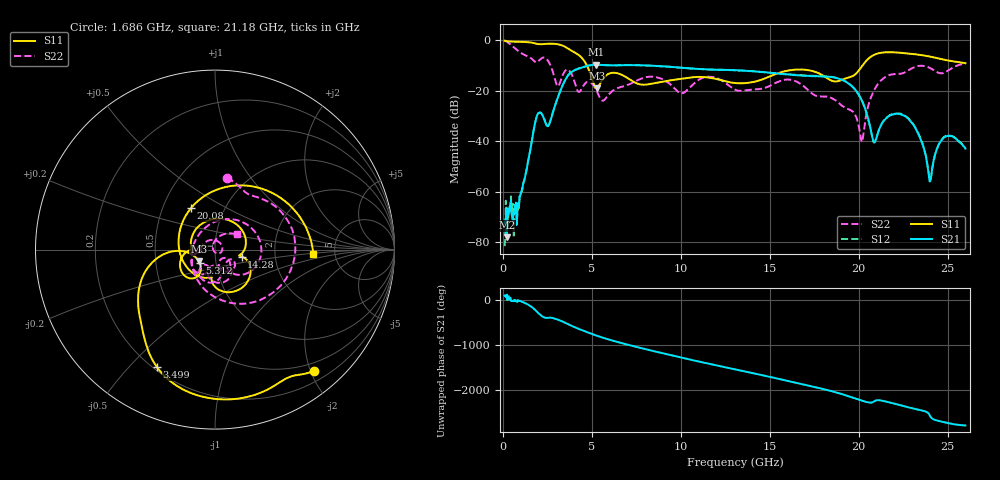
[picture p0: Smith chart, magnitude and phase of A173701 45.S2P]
!  2-Port S-parameters saved by WinCal
! VAR MeasName=S-Parameters (CALIBRATED_DATA) read from VNA (N5245A)
! VAR MeasDate=2017-6-7 10:31:25
! VAR NAME=A173701 45
! VAR FILENAME=A173701 45.S2P
! VAR DATE=2017-6-7 10:31:25
! VAR PHYS_PORTS=1,2
# Hz S DB R 50
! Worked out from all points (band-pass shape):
!   801 points, 100 MHz to 26 GHz, reference 50 ohm
!   highest |S21| = -9.82 dB at 5.248 GHz (marker M1); lowest = -78.0 dB at 229.5 MHz (marker M2)
!   |S21| within 3 dB of the highest: 3.837 GHz to 14.77 GHz (10.93 GHz wide, 118 % of centre)
!   lowest |S11| = -19.1 dB at 5.28 GHz (marker M3), VSWR 1.25, Z = 41.4 - j5.43 ohm
!   |S11| at or under -10 dB: 4.715 GHz to 20.23 GHz (15.51 GHz wide, 124 % of centre)
!   |S22| runs from -40.4 to -0.2 dB; largest |S21 - S12| = 0.0049
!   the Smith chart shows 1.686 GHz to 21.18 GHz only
!   S11 on the Smith chart (normalised r, x): 1.686 GHz: 0.36, -2.05; 3.499 GHz: 0.21, -0.60; 5.312 GHz: 0.83, -0.12; 14.28 GHz: 1.34, -0.11; 20.08 GHz: 0.69, +0.34; 21.18 GHz: 3.42, -0.26
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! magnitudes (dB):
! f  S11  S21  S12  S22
! 100 MHz  -0.3  -72.5  -81.5  -0.2
! 229.5 MHz  -0.6  -78.0  -70.0  -0.7
! 909.4 MHz  -0.8  -65.7  -66.4  -4.6
! 1.686 GHz  -1.2  -37.5  -37.5  -7.8
! 2.593 GHz  -1.5  -33.6  -33.6  -8.9
! 3.499 GHz  -2.7  -16.0  -15.9  -12.3
! 4.438 GHz  -7.1  -10.9  -10.9  -19.2
! 5.248 GHz  -19.1  -9.8  -9.8  -19.8
! 5.28 GHz  -19.1  -9.8  -9.8  -20.2
! 5.312 GHz  -18.9  -9.8  -9.8  -20.7
! 8.744 GHz  -16.8  -10.3  -10.4  -14.9
! 13.05 GHz  -17.0  -12.0  -12.0  -19.7
! 14.28 GHz  -16.3  -12.5  -12.5  -19.5
! 17.39 GHz  -12.3  -14.3  -14.2  -21.2
! 20.08 GHz  -11.5  -22.5  -22.6  -36.5
! 20.82 GHz  -6.1  -39.9  -40.1  -20.6
! 21.18 GHz  -5.2  -34.9  -34.8  -16.6
! 21.69 GHz  -4.9  -30.1  -30.0  -14.0
! 23.05 GHz  -5.6  -33.4  -33.1  -11.0
! 23.99 GHz  -6.6  -55.9  -55.4  -11.0
! 24.83 GHz  -7.9  -38.5  -38.1  -12.9
! 26 GHz  -9.2  -42.9  -42.8  -9.5
